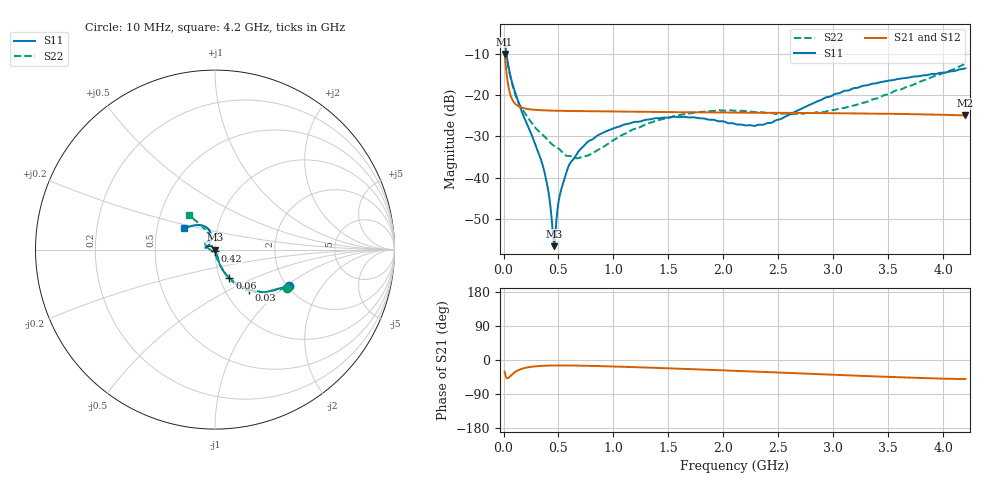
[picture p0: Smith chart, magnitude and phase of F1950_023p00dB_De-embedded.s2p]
! Integrated Device Technology
! Corporate Headquarters
! 6024 Silver Creek Valley Road
! San Jose, CA 95138  USA
! Phone:  1-408-284-8200
! Toll Free:  1-800-223-1366
! Webpage:  http://www.idt.com/
! Timing and RF Division
! 515 Groton Road, Suite 102
! Westford, MA 01886-6024
! Device:  F1950
! Description: 7-bit 0.25 dB Digital Step Attenuator
! Frequency:  150.0 -  4000.00 MHz
! Package:  4x4 mm Thin QFN Plastic Package: 24 pin
! Ports:  2 RF, 12 DC
!  Pin  1  = D0
!  Pin  2  = VDD
!  Pin  3  = Vmode
!  Pin  4  = GND
!  Pin  5  = RF1  =  Port 1
!  Pin  6  = GND
!  Pin  7  = GND
!  Pin  8  = GND
!  Pin  9  = GND
!  Pin 10  = GND
!  Pin 11  = GND
!  Pin 12  = GND
!  Pin 13  = GND
!  Pin 14  = RF2  =  Port 2
!  Pin 15  = GND
!  Pin 16  = LE
!  Pin 17  = CLK
!  Pin 18  = DATE
!  Pin 19  = D6
!  Pin 20  = D5
!  Pin 21  = D4
!  Pin 22  = D3
!  Pin 23  = D2
!  Pin 24  = D1
! State:  92
! Atten State:  23.00 dB
! Voltage:  +5.00 Volts
! Current:  Not Measured mA
! Data:  The device was measured on a the F195X evaluation board which has
!  individual transmission lines to the RF pins.  Data was collected
!  using a calibrated network analyzer.  The evaluation board was
!  de-embedded using a TRL calibration technique.
!  The reference plane is the edge of the package pin.
! Misc:  Board 2019
!  Action Tracker AT0250
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# GHz S dB R 50
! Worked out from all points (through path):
!   420 points, 10 MHz to 4.2 GHz, reference 50 ohm
!   highest |S21| = -9.99 dB at 10 MHz (marker M1); lowest = -24.9 dB at 4.2 GHz (marker M2)
!   group delay of S21, straight-line fit = 23.8 ps
!   lowest |S11| = -56.7 dB at 460 MHz (marker M3), VSWR 1.00, Z = 49.9 - j0.0693 ohm
!   |S11| at or under -10 dB: 26.65 MHz to end of sweep
!   |S22| runs from -35.3 to -6.9 dB; largest |S21 - S12| = 0.00011
!   S11 on the Smith chart (normalised r, x): 10 MHz: 2.06, -1.05; 30 MHz: 1.29, -0.64; 60 MHz: 1.11, -0.36; 420 MHz: 1.00, -0.01; 4.2 GHz: 0.69, +0.17
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0.01  -6.73 -25.9  -9.99 -31.1  -9.99 -31.1  -6.86 -28.2
0.03  -10.63 -49.7  -15.30 -47.9  -15.30 -47.8  -10.99 -52.0
0.06  -15.02 -63.1  -19.70 -43.1  -19.70 -43.1  -15.24 -64.5
0.1  -18.89 -70.0  -21.91 -32.9  -21.91 -32.9  -19.28 -69.8
0.15  -22.84 -72.0  -22.88 -25.1  -22.88 -25.1  -22.49 -73.9
0.35  -36.46 -69.3  -23.68 -15.5  -23.67 -15.5  -29.43 -84.4
0.39  -40.85 -71.1  -23.72 -15.0  -23.72 -15.0  -30.52 -85.9
0.42  -45.52 -80.1  -23.75 -14.7  -23.75 -14.7  -31.38 -88.0
0.44  -50.56 -93.4  -23.76 -14.6  -23.76 -14.6  -31.92 -91.0
0.46  -56.66 -151.8  -23.78 -14.5  -23.77 -14.5  -32.33 -94.4
0.48  -50.72 150.9  -23.79 -14.4  -23.79 -14.4  -32.63 -97.4
0.51  -44.51 139.9  -23.81 -14.4  -23.81 -14.4  -33.16 -100.2
0.57  -38.93 134.6  -23.84 -14.4  -23.83 -14.4  -34.68 -111.0
0.71  -32.85 137.6  -23.89 -15.0  -23.89 -15.0  -35.02 -139.5
0.95  -28.59 146.0  -23.97 -16.7  -23.97 -16.7  -31.81 -176.6
1.41  -25.59 162.7  -24.10 -21.0  -24.10 -21.1  -26.06 160.8
1.73  -25.39 168.1  -24.16 -24.3  -24.16 -24.3  -24.24 152.5
2.11  -27.04 157.6  -24.23 -28.7  -24.23 -28.8  -23.80 142.7
2.43  -26.74 126.0  -24.29 -32.1  -24.29 -32.1  -24.37 132.0
2.81  -22.07 105.2  -24.35 -36.7  -24.35 -36.7  -24.35 116.7
3.51  -16.45 117.2  -24.52 -44.6  -24.52 -44.6  -19.67 113.4
4.2  -13.50 145.5  -24.93 -50.3  -24.93 -50.4  -12.42 127.1
